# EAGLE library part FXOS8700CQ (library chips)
Accelerometer, Magnetometer, 3 Axis Sensor, I2C/SPI
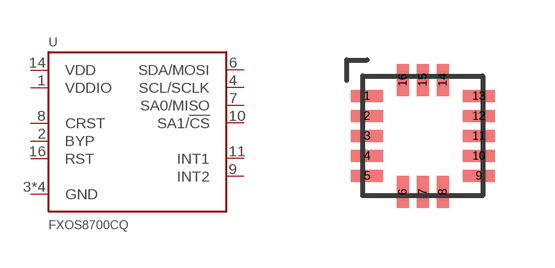
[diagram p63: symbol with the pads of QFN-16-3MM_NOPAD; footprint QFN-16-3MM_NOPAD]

Designator prefix U

## FXOS8700CQ (DIGIKEY: FXOS8700CQR1CT-ND; MPN: FXOS8700CQR1)  [QFN-16-3MM_NOPAD]
1  VDDIO
2  BYP
3  GND
4  SCL/SCLK
5  GND
6  SDA/MOSI
7  SA0/MISO
8  CRST
9  INT2
10  SA1/!CS
11  INT1
12  GND
13  GND
14  VDD
16  RST

## Footprint QFN-16-3MM_NOPAD (pad centres in mm)
smd 0.8 x 0.3: 1 -1.4,1; 2 -1.4,0.5; 3 -1.4,0; 4 -1.4,-0.5; 5 -1.4,-1; 9 1.4,-1; 10 1.4,-0.5; 11 1.4,0; 12 1.4,0.5; 13 1.4,1
smd 0.3 x 0.8: 6 -0.5,-1.4; 7 0,-1.4; 8 0.5,-1.4; 14 0.5,1.4; 15 0,1.4; 16 -0.5,1.4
